(* Logix 5000 DataType export R4AO8DIDO_Seneca_InData; software revision 35.00 *)

TYPE R4AO8DIDO_Seneca_InData :   // User Define Measure Data Type for Seneca R-4AO-8DIDO-E Device
STRUCT
   DIN1 : BOOL;
   DIN2 : BOOL;
   DIN3 : BOOL;
   DIN4 : BOOL;
   DIN5 : BOOL;
   DIN6 : BOOL;
   DIN7 : BOOL;
   DIN8 : BOOL;
   COUNT1 : UDINT;
   COUNT2 : UDINT;
   COUNT3 : UDINT;
   COUNT4 : UDINT;
   COUNT5 : UDINT;
   COUNT6 : UDINT;
   COUNT7 : UDINT;
   COUNT8 : UDINT;
   FREQ1 : REAL;
   FREQ2 : REAL;
   FREQ3 : REAL;
   FREQ4 : REAL;
   FREQ5 : REAL;
   FREQ6 : REAL;
   FREQ7 : REAL;
   FREQ8 : REAL;
   FLAGS : INT;
END_STRUCT
END_TYPE
